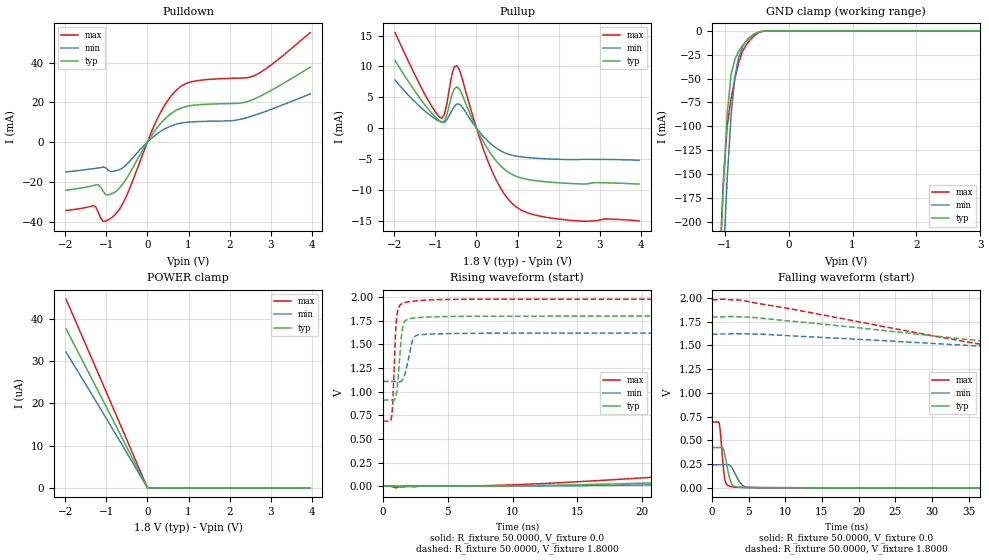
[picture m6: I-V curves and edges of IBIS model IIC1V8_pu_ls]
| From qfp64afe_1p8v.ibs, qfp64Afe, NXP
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[Model] IIC1V8_pu_ls
|   Model IIC1V8_pu_ls
| This model was characterised for following simulation conditions:
| External (pad) voltage:
|   - Typ: 1.8V,   - Min: 1.62V,   - Max: 1.98V
| Library cells for typ/min/max conditions are connected as defined below:
|  IO - External Pad
|  A - Core Input
|  EN - Output Buffer Enable
|  BOOST - vdde
|  EGP - vdd
|  EHS - gnd
|  ENZI - vdd
|  EPD - gnd
|  EPUN - gnd
|  ZI - NC
|  ZIF - NC
|  gnd - gnd
|  gnde - gnde
|  vdd - vdd
|  vdde - vdde
| All other pins connected to ground
Model_type I/O
Polarity   Non-Inverting
Enable   Active-Low
Vinl =   0.5400V
Vinh =   1.2600V
Vmeas =  0.9000V
Cref =   0.0F
Rref =   1.0000k
Vref =   0.0V
C_comp   3.6100pF   3.4623pF   3.7513pF
|C_comp_pullup   0.9280pF   0.9063pF   0.9342pF
|C_comp_pulldown   2.3312pF   2.4847pF   2.1853pF
[Model Spec]
| variable   typ   min   max
Vinh   0.5400V   0.4860V   0.5940V
Vinl   1.2600V   1.1340V   1.3860V
Vmeas   0.9000V   0.8100V   0.9900V
[Temperature Range]   25.0000   0.1250k   -40.0000
[Voltage Range]   1.8000V   1.6200V   1.9800V
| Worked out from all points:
|   slope of the pulldown table from 0 to 0.27 V, typ, clamps not added: 33.4 ohm
|   slope of the pullup table from 0 to 0.27 V, typ, clamps not added: 80.7 ohm
|   GND clamp passes 1 mA (typ) near -0.44 V on its own axis
|   rising waveform, R_fixture 50.0000, V_fixture 0.0: 20-80 % time 70.1ns typ, 81.9ns min, 57ns max; typ from 0.001 V to 0.424 V
|   rising waveform, R_fixture 50.0000, V_fixture 1.8000: 20-80 % time 318ps typ, 486ps min, 235ps max; typ from 0.912 V to 1.8 V
|   falling waveform, R_fixture 50.0000, V_fixture 0.0: 20-80 % time 673ps typ, 1.04ns min, 475ps max; typ from 0.424 V to 0.001 V
|   falling waveform, R_fixture 50.0000, V_fixture 1.8000: 20-80 % time 66.9ns typ, 88.7ns min, 49ns max; typ from 1.8 V to 0.912 V
[Pulldown]
|Voltage   I(typ)   I(min)   I(max)
-1.98V    -24.22mA   -15.04mA   -34.42mA
-1.32V    -21.94mA   -13.4mA    -32.06mA
-1.2V     -21.45mA   -13.05mA   -35.06mA
-1.08V    -24.63mA   -12.6mA    -39.9mA
-900mV    -26.23mA   -14.78mA   -38.53mA
-720mV    -24.07mA   -14.13mA   -34.99mA
-540mV    -19.33mA   -11.9mA    -28.53mA
300mV     8.856mA    5.096mA    14.12mA
720mV     16.26mA    9.117mA    26.48mA
1.14V     18.6mA     10.26mA    30.69mA
2.58V     21.55mA    13.34mA    33.32mA
3.96V     37.7mA     24.26mA    55.17mA
[Pullup]
|Voltage   I(typ)   I(min)   I(max)
-1.98V    10.93mA    7.779mA    15.48mA
-1.26V    3.804mA    2.797mA    5.531mA
-840mV    976.5uA    916.9uA    1.58mA
-720mV    2.123mA    1.339mA    3.886mA
-600mV    5.282mA    2.828mA    8.607mA
-480mV    6.665mA    3.904mA    10.12mA
-420mV    6.371mA    3.888mA    9.538mA
360mV     -4.265mA   -2.608mA   -6.666mA
660mV     -6.57mA    -3.917mA   -10.5mA
960mV     -7.8mA     -4.537mA   -12.74mA
2.04V     -8.889mA   -5.075mA   -14.77mA
3.96V     -9.081mA   -5.209mA   -15.04mA
[GND_clamp]
|Voltage   I(typ)   I(min)   I(max)
-1.98V    -2.104A    -2.075A    -2.136A
-1.08V    -259.3mA   -333mA     -247mA
-1.02V    -161.8mA   -238.7mA   -157.2mA
-960mV    -86.78mA   -154.8mA   -99.51mA
-900mV    -45.99mA   -88.85mA   -71.1mA
-840mV    -29.94mA   -48.03mA   -50.31mA
-780mV    -21.2mA    -27.67mA   -33.04mA
-720mV    -15.2mA    -16.91mA   -21.32mA
-660mV    -10.61mA   -10.27mA   -14.61mA
-540mV    -3.83mA    -3.432mA   -5.346mA
-300mV    -56.31uA   -67.68uA   -68.13uA
3.96V     0A         0A         0A
[POWER_clamp]
|Voltage   I(typ)   I(min)   I(max)
-1.98V    37.59uA    32.11uA    44.63uA
-960mV    18.36uA    15.76uA    21.73uA
0V        104.7pA    4.893nA    11.38pA
3.96V     0A         0A         0A
[Ramp]
| variable   typ   min   max
dV/dt_r  0.2543/70.1044n   0.1459/81.9484n   0.4154/57.0287n
dV/dt_f  0.5329/66.9322n   0.3063/88.6823n   0.7748/48.9625n
R_load = 50.0000
[Rising Waveform]
R_fixture= 50.0000
V_fixture= 0.0
V_fixture_min= 0.0
V_fixture_max= 0.0
|time   V(typ)   V(min)   V(max)
0s        634.5uV    668.6uV    603.2uV
1.012ns   -2.646mV   860.1uV    -18.46mV
1.63ns    -9.938mV   -2.025mV   404.7uV
12.66ns   7.947mV    2.714mV    29.16mV
45.92ns   147.1mV    66.25mV    307mV
84.46ns   286.5mV    144.5mV    562.7mV
103.3ns   341.3mV    173.2mV    630.8mV
133.9ns   393.5mV    209mV      673.9mV
250.5ns   423.6mV    242.4mV    692.6mV
1us       424.5mV    243.9mV    693mV
[Rising Waveform]
R_fixture= 50.0000
V_fixture= 1.8000
V_fixture_min= 1.6200
V_fixture_max= 1.9800
|time   V(typ)   V(min)   V(max)
0s        911.7mV    1.109V     688.6mV
685.4ps   910.1mV    1.109V     746mV
787.2ps   907.8mV    1.11V      947.4mV
1.008ns   952.1mV    1.108V     1.695V
1.269ns   1.305V     1.105V     1.905V
1.479ns   1.64V      1.118V     1.933V
1.768ns   1.756V     1.218V     1.947V
2.477ns   1.781V     1.585V     1.961V
5.33ns    1.797V     1.616V     1.977V
1us       1.8V       1.62V      1.98V
[Falling Waveform]
R_fixture= 50.0000
V_fixture= 0.0
V_fixture_min= 0.0
V_fixture_max= 0.0
|time   V(typ)   V(min)   V(max)
0s        424.5mV    243.9mV    693mV
1.011ns   424.5mV    243.9mV    675.6mV
1.155ns   425.8mV    243.9mV    586.9mV
1.623ns   399.4mV    244mV      166.6mV
1.944ns   280.7mV    245.5mV    46.11mV
2.413ns   103.5mV    240.5mV    18.41mV
2.833ns   27.24mV    201.3mV    11.35mV
4.002ns   6.158mV    41.61mV    5.38mV
5.073ns   3.509mV    6.241mV    4.024mV
1us       634.5uV    668.7uV    603.2uV
[Falling Waveform]
R_fixture= 50.0000
V_fixture= 1.8000
V_fixture_min= 1.6200
V_fixture_max= 1.9800
|time   V(typ)   V(min)   V(max)
0s        1.8V       1.62V      1.98V
4.134ns   1.8V       1.623V     1.974V
57.87ns   1.395V     1.407V     1.247V
67.63ns   1.332V     1.373V     1.008V
75.59ns   1.28V      1.347V     876.9mV
89.98ns   1.132V     1.304V     769.2mV
112.4ns   990.3mV    1.235V     713.6mV
149.4ns   929.1mV    1.143V     693.1mV
209.7ns   914mV      1.114V     689.1mV
1us       911.8mV    1.109V     688.6mV
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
